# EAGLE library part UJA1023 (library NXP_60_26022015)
LIN-I/O slave The UJA1023 is a stand-alone Local Interconnect Network (LIN) I/O slave that replaces basic components commonly used in electronic control units for input and output handling. The UJA1023 contains a LIN 2.0 controller, an integrated LIN transceiver which is LIN 2.0 / SAE J2602 compliant and LIN 1.3 compatible, a 30 kΩ termination resistor necessary for LIN-slaves, and eight I/O ports which are configurable via the LIN bus. An automatic bit rate synchronization circuit adapts to any (master) bit rate between 1 kbit/s and 20 kbit/s. For this, an oscillator is integrated. The LIN protocol will be handled autonomously and both Node Address (NAD) and LIN frame Identifier (ID) programming will be done by a master request and an optional slave response message in combination with a daisy chain or plug coding function. AAL Eindhoven MK
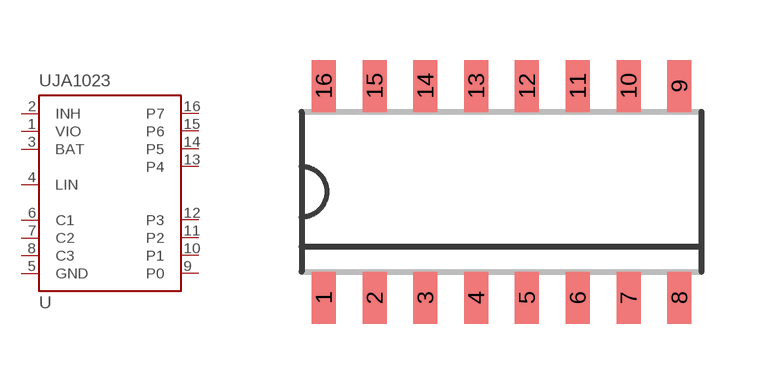
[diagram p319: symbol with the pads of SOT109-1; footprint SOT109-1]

Designator prefix U

## UJA1023T  [SOT109-1]
1  VIO  pwr
2  INH  out
3  BAT  pwr
4  LIN
5  GND  pwr
6  C1  in
7  C2  in
8  C3
9  P0
10  P1
11  P2
12  P3
13  P4
14  P5
15  P6
16  P7

## Footprint SOT109-1 (pad centres in mm)
SOT109-1 SO16: plastic small outline package; 16 leads; body width 3.9 mm JEDEC: MS-012 IEC: 076E07
smd 0.6 x 1.3: 1 -4.445,-2.65; 2 -3.175,-2.65; 3 -1.905,-2.65; 4 -0.635,-2.65; 5 0.635,-2.65; 6 1.905,-2.65; 7 3.175,-2.65; 8 4.445,-2.65; 9 4.445,2.65; 10 3.175,2.65; 11 1.905,2.65; 12 0.635,2.65; 13 -0.635,2.65; 14 -1.905,2.65; 15 -3.175,2.65; 16 -4.445,2.65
